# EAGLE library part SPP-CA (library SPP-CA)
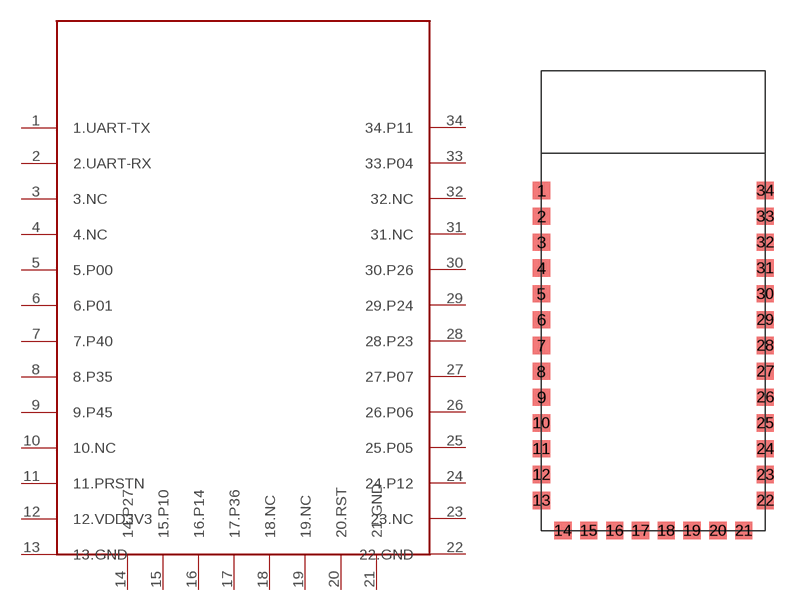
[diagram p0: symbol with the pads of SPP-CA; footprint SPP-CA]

Designator prefix -

## SPP-CA  [SPP-CA]
1  1.UART-TX
2  2.UART-RX
3  3.NC
4  4.NC
5  5.P00
6  6.P01
7  7.P40
8  8.P35
9  9.P45
10  10.NC
11  11.PRSTN
12  12.VDD3V3
13  13.GND
14  14.P27
15  15.P10
16  16.P14
17  17.P36
18  18.NC
19  19.NC
20  20.RST
21  21.GND
22  22.GND
23  23.NC
24  24.P12
25  25.P05
26  26.P06
27  27.P07
28  28.P23
29  29.P24
30  30.P26
31  31.NC
32  32.NC
33  33.P04
34  34.P11

## Footprint SPP-CA (pad centres in mm)
smd 1 x 1: 1 0,19.75; 2 0,18.25; 3 0,16.75; 4 0,15.25; 5 0,13.75; 6 0,12.25; 7 0,10.75; 8 0,9.25; 9 0,7.75; 10 0,6.25; 11 0,4.75; 12 0,3.25; 13 0,1.75; 14 1.25,0; 15 2.75,0; 16 4.25,0; 17 5.75,0; 18 7.25,0; 19 8.75,0; 20 10.25,0; 21 11.75,0; 22 13,1.75; 23 13,3.25; 24 13,4.75; 25 13,6.25; 26 13,7.75; 27 13,9.25; 28 13,10.75; 29 13,12.25; 30 13,13.75; 31 13,15.25; 32 13,16.75; 33 13,18.25; 34 13,19.75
